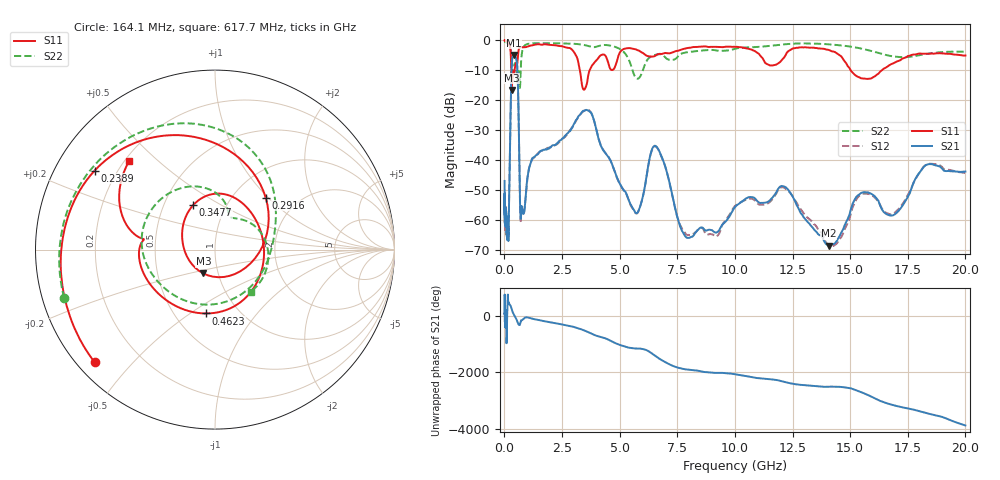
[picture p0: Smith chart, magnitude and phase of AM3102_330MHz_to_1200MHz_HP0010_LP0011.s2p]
! Date/Time: Tue, Sep 11, 2018 5:10 PM
! Network Analyzer: Agilent Technologies E8362B Rev: A.07.50.63
! Sweep from 0.010 to 20.000 GHz, 1601 Points, Sweep Type: LOG
! Power Supply: 4.950 V, 0.001 A
# Hz S DB R 50
!freq MagS11 AngS11 MagS21 AngS21 MagS12 AngS12 MagS22 AngS22
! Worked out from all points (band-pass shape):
!   1601 points, 10 MHz to 20 GHz, reference 50 ohm
!   highest |S21| = -4.82 dB at 410.6 MHz (marker M1); lowest = -68.7 dB at 14.07 GHz (marker M2)
!   |S21| within 3 dB of the highest: 322 MHz to 549 MHz (227 MHz wide, 52.1 % of centre)
!   lowest |S11| = -16.6 dB at 319.2 MHz (marker M3), VSWR 1.35, Z = 42.5 - j11.5 ohm
!   |S11| at or under -10 dB: 297.8 MHz to 438.4 MHz (140.6 MHz wide, 38.2 % of centre); 3.276 GHz to 3.697 GHz (421.3 MHz wide, 12.1 % of centre); 15.03 GHz to 16.37 GHz (1.349 GHz wide, 8.59 % of centre)
!   |S22| runs from -15.9 to -0.2 dB; largest |S21 - S12| = 0.013
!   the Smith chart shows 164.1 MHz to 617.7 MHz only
!   S11 on the Smith chart (normalised r, x): 164.1 MHz: 0.05, -0.39; 238.9 MHz: 0.12, +0.29; 291.6 MHz: 1.40, +0.97; 347.7 MHz: 0.70, +0.37; 462.3 MHz: 0.71, -0.58; 617.7 MHz: 0.22, +0.41
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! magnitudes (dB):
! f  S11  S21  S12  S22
! 10 MHz  0.0  -47.0  -51.9  -0.2
! 35.55 MHz  0.0  -59.9  -60.3  -0.4
! 126.4 MHz  -0.4  -63.2  -62.4  -0.9
! 164.1 MHz  -0.7  -63.8  -64.7  -1.1
! 238.9 MHz  -1.9  -38.5  -38.5  -1.9
! 291.6 MHz  -7.9  -15.3  -15.4  -4.3
! 319.2 MHz  -16.6  -8.2  -8.2  -8.1
! 347.7 MHz  -11.2  -5.9  -5.9  -10.7
! 410.6 MHz  -11.3  -4.8  -4.9  -8.8
! 447.2 MHz  -9.5  -5.1  -5.1  -7.7
! 462.3 MHz  -8.9  -5.3  -5.3  -7.6
! 556.4 MHz  -7.8  -8.5  -8.7  -13.9
! 617.7 MHz  -3.2  -25.4  -25.5  -10.2
! 705.6 MHz  -2.2  -59.5  -60.5  -10.9
! 1.59 GHz  -1.4  -36.9  -36.9  -0.9
! 3.651 GHz  -11.2  -23.5  -23.3  -1.9
! 5.652 GHz  -2.9  -57.3  -57.4  -11.9
! 6.58 GHz  -4.9  -35.4  -35.6  -4.8
! 7.92 GHz  -2.6  -66.1  -65.1  -4.0
! 12.09 GHz  -6.1  -48.8  -49.1  -1.3
! 14.07 GHz  -3.2  -68.7  -68.5  -1.3
! 20 GHz  -5.0  -43.9  -44.4  -3.8
